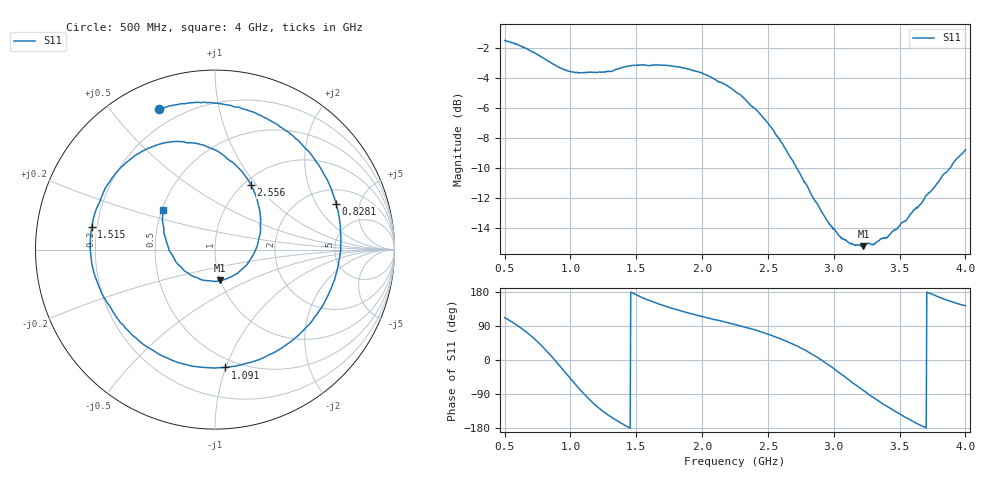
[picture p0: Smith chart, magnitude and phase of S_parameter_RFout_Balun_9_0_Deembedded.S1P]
!Agilent Technologies,E5071B,MY42403504,A.06.51
!Date: Wed Feb 26 14:57:02 2014
!Data & Calibration Information:
!Freq	S11:SOLT1(ON)
# Hz S dB R 50
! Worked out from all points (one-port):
!   801 points, 500 MHz to 4 GHz, reference 50 ohm
!   lowest |S11| = -15.2 dB at 3.226 GHz (marker M1), VSWR 1.42, Z = 49.8 - j17.6 ohm
!   |S11| at or under -10 dB: 2.718 GHz to 3.883 GHz (1.165 GHz wide, 35.3 % of centre)
!   S11 on the Smith chart (normalised r, x): 500 MHz: 0.12, +0.67; 828.1 MHz: 2.82, +2.99; 1.091 GHz: 0.43, -0.99; 1.515 GHz: 0.18, +0.09; 2.556 GHz: 1.08, +0.93; 4 GHz: 0.51, +0.25
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5e8  -1.47 111.8
5.91875e8  -1.72 92.2
6.75e8  -2.05 71.0
7.49375e8  -2.43 48.4
8.28125e8  -2.84 20.6
8.85e8  -3.12 -1.6
9.375e8  -3.36 -23.2
1.01625e9  -3.57 -55.9
1.090625e9  -3.63 -85.0
1.1475e9  -3.59 -105.4
1.22625e9  -3.59 -129.6
1.291875e9  -3.53 -146.6
1.375e9  -3.34 -164.6
1.515e9  -3.10 169.6
1.668125e9  -3.11 148.2
1.8125e9  -3.24 132.1
2.0225e9  -3.75 112.8
2.25e9  -4.86 93.5
2.420625e9  -6.19 77.5
2.55625e9  -7.71 61.1
2.6875e9  -9.50 42.1
2.884375e9  -12.54 5.0
3.125e9  -15.05 -55.2
3.225625e9  -15.22 -80.6
3.365625e9  -14.72 -114.1
3.5625e9  -13.37 -154.3
3.820625e9  -10.57 163.2
4e9  -8.78 143.2
